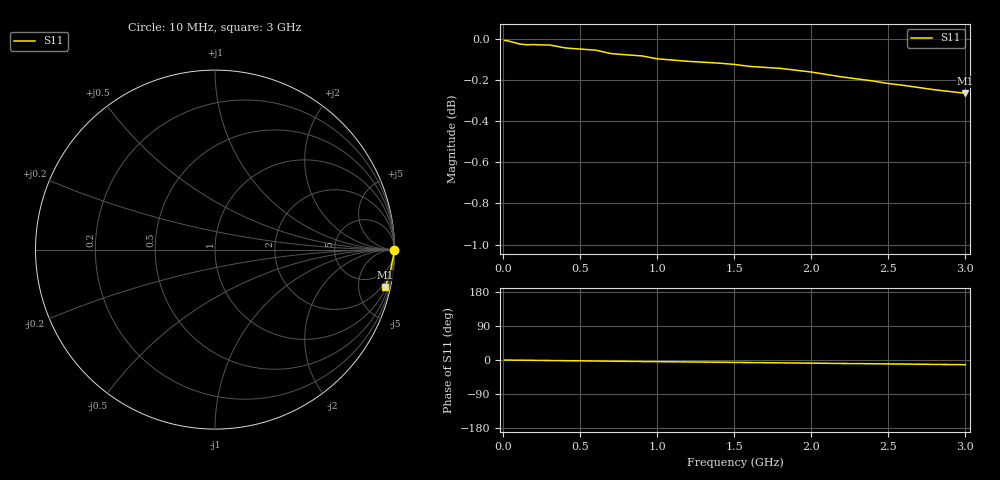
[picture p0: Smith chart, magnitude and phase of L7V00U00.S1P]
! SIEMENS Small Signal Semiconductors
! BAR14-1
! Si PIN Diode in SOT23
! VR = 0 V
! S-Parameters:  July  1992
# GHz  S  MA  R  50
!  f  S11
! GHz  MAG  ANG
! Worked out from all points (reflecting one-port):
!   31 points, 10 MHz to 3 GHz, reference 50 ohm
!   lowest |S11| = -0.3 dB at 3 GHz (marker M1), VSWR 65.67, Z = 64 - j451 ohm
!   phase of S11 starts at -0 deg and turns -12 deg over the sweep
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0.01  0.9991 -0.1
0.05  0.9984 -0.3
0.06  0.9982 -0.4
0.08  0.9978 -0.4
0.1  0.9972 -0.5
0.15  0.9967 -0.7
0.2  0.9968 -0.9
0.25  0.9966 -1.1
0.3  0.9966 -1.4
0.4  0.995 -1.8
0.5  0.9943 -2.2
0.6  0.9937 -2.7
0.7  0.9918 -3.1
0.8  0.9911 -3.5
0.9  0.9905 -3.9
1  0.9889 -4.3
1.2  0.9875 -5.1
1.4  0.9865 -5.9
1.5  0.9858 -6.3
1.6  0.9847 -6.7
1.8  0.9836 -7.5
2  0.9816 -8.3
2.2  0.9789 -9.2
2.4  0.9767 -9.9
2.5  0.9753 -10.4
2.6  0.9743 -10.7
2.8  0.9719 -11.6
3  0.97 -12.4
